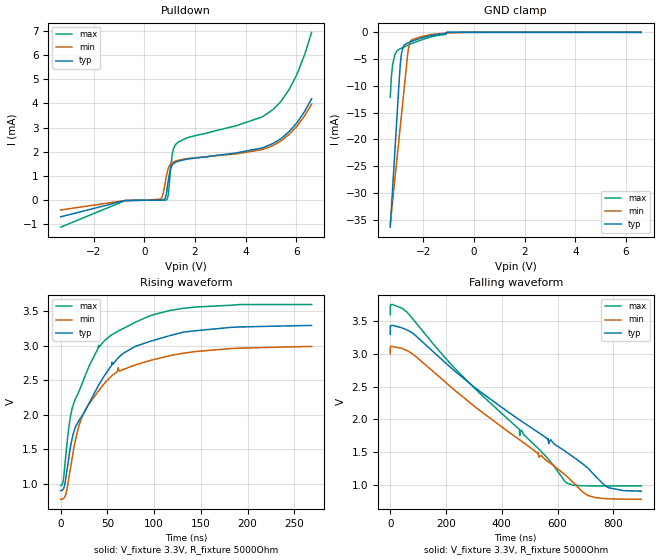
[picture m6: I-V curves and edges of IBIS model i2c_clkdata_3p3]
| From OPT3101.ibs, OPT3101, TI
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|   i2c_clkdata_3p3 Model
[Model]   i2c_clkdata_3p3
Model_type   I/O_open_drain
Polarity   Inverting
Vinl = 0.99
Vinh = 2.31
Vmeas = 1.65
Vref = 3.3
Cref = 2pF
Rref = 5000
|   typ   min   max
|   (nom PVT)   (fast PVT)   (slow PVT)
C_comp   1.487e-12   1.014e-12   1.822e-12
[Model spec]
|subparameter
Vinl   0.99   0.90   1.08
Vinh   2.31   2.10   2.52
| Where nom  PVT is Nominal Process, 3.3V, 27C
|   Fast PVT is Strong Process,  3.6V, -40C
|   Slow PVT is Weak Process,   3V, 125C
[Voltage Range]   3.3   3   3.6
|Junction Temperature
[Temperature Range]   27   125   -40
[Pullup Reference]   3.3   3   3.6
[Pulldown Reference]   0   0   0
[Power Clamp Reference]   3.3   3   3.6
[GND Clamp Reference]   0   0   0
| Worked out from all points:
|   falling waveform, V_fixture 3.3V, R_fixture 5000Ohm: 20-80 % time 461ns typ, 406ns min, 373ns max; typ from 3.3 V to 0.901 V
|   rising waveform, V_fixture 3.3V, R_fixture 5000Ohm: 20-80 % time 52.3ns typ, 42.9ns min, 40.8ns max; typ from 0.901 V to 3.29 V
[Pulldown]
|   Voltage   I(typ)   I(min)   I(max)
-3.3V     -684.7uA   -402.2uA   -1.112mA
-751.2mV  -10.66uA   -10.49uA   -14.64uA
652.8mV   189.7nA    45.25uA    223.6pA
818.4mV   74.31uA    694.2uA    1.079uA
879mV     330.3uA    1.041mA    19.26uA
950.4mV   851.2uA    1.336mA    289.1uA
1.109V    1.469mA    1.561mA    1.941mA
1.251V    1.574mA    1.623mA    2.319mA
5.074V    2.341mA    2.259mA    3.744mA
5.409V    2.559mA    2.462mA    4.109mA
6.006V    3.183mA    3.042mA    5.17mA
6.6V      4.194mA    3.968mA    6.935mA
[GND Clamp]
|   Voltage   I(typ)   I(min)   I(max)
-3.3V     -36.4mA    -35.87mA   -12.12mA
-3.255V   -32.9mA    -33.79mA   -8.337mA
-3.204V   -28.96mA   -31.44mA   -6.012mA
-3.124V   -22.68mA   -27.71mA   -4.221mA
-2.897V   -5.586mA   -17.25mA   -3.065mA
-2.795V   -2.792mA   -12.52mA   -2.825mA
-2.716V   -2.264mA   -8.856mA   -2.648mA
-2.623V   -2.029mA   -4.584mA   -2.451mA
-2.541V   -1.853mA   -2.114mA   -2.281mA
-1.982V   -921uA     -689uA     -1.269mA
-1.1V     -220.7uA   -148.9uA   -6.034uA
6.6V      0A         0A         0A
[POWER Clamp]
|   Voltage   I(typ)   I(min)   I(max)
-3.3V     0A         0A         0A
0V        0A         0A         0A
6.6V      0A         0A         0A
[Ramp]
R_load = 5000
|   typ   min   max
dV/dt_r   1.43899/5.27535e-08   1.33369/4.36471e-08   1.57511/4.10469e-08
dV/dt_f   1.43941/4.61445e-07   1.33431/4.06144e-07   1.57108/3.73189e-07
[Falling Waveform]
V_fixture = 3.3V
V_fixture_min = 3V
V_fixture_max = 3.6V
R_fixture = 5000Ohm
|   Time   V(typ)   V(min)   V(max)
0s        3.3V       3V         3.6V
500ps     3.423V     3.099V     3.744V
5.6ns     3.433V     3.111V     3.753V
58.6ns    3.366V     3.052V     3.643V
321.9ns   2.424V     2.131V     2.393V
470.4ns   1.971V     1.666V     1.833V
635ns     1.488V     1.12V      1.021V
706.8ns   1.26V      839.3mV    982.1mV
782.1ns   953.7mV    784.6mV    980.8mV
899.9ns   901mV      776.1mV    981.5mV
[Rising Waveform]
V_fixture = 3.3V
V_fixture_min = 3V
V_fixture_max = 3.6V
R_fixture = 5000Ohm
|   Time   V(typ)   V(min)   V(max)
0s        900.9mV    776mV      974.3mV
2.7ns     921mV      784.7mV    1.04V
5.9ns     1.12V      869.5mV    1.476V
13.3ns    1.716V     1.463V     2.138V
27ns      2.076V     2.087V     2.59V
40.5ns    2.425V     2.344V     3.003V
53.3ns    2.691V     2.546V     3.143V
79.6ns    2.986V     2.719V     3.335V
131.1ns   3.195V     2.889V     3.538V
268.5ns   3.29V      2.987V     3.594V
